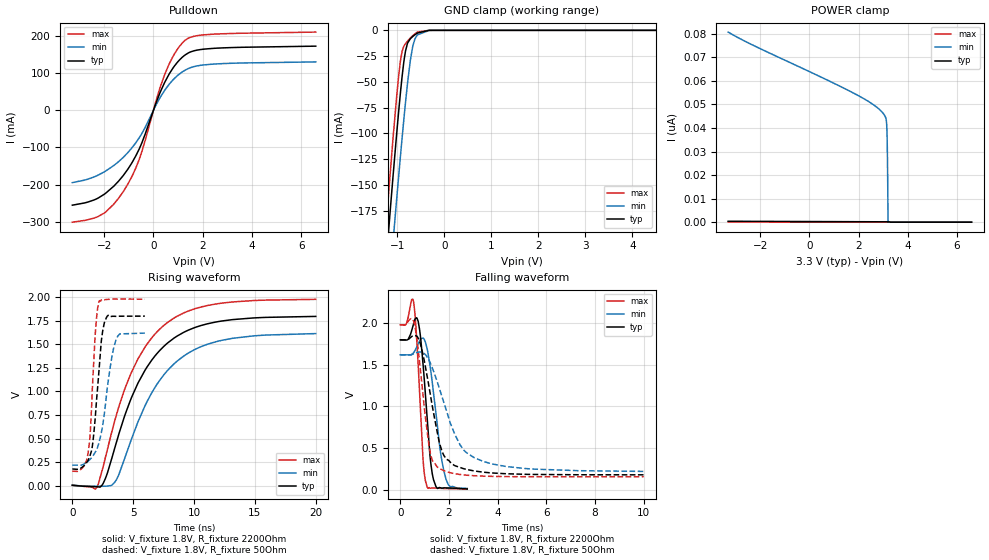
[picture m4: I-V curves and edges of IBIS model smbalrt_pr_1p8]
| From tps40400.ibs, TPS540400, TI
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|   smbalrt_pr_1p8 Model
[Model]   smbalrt_pr_1p8
Model_type   Open_sink
Polarity   Inverting
Vmeas = 1.65
Vref = 3.3
Cref = 2pF
Rref = 2200
|   typ   min   max
|   (nom PVT)   (fast PVT)   (slow PVT)
C_comp   1.150e-12   1.129e-12   1.173e-12
| Where nom  PVT is Nominal Process, 3.3V, 25C
|   Fast PVT is Strong Process,  3.4V, -40C
|   Slow PVT is Weak Process,   3.2V, 125C
[Voltage Range]   3.3   3.2   3.4
|Junction Temperature
[Temperature Range]   25   125   -40
[Pullup Reference]   3.3   3.2   3.4
[Pulldown Reference]   0   0   0
[Power Clamp Reference]   3.3   3.2   3.4
[GND Clamp Reference]   0   0   0
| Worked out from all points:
|   slope of the pulldown table from 0 to 0.495 V, typ, clamps not added: 6.2 ohm
|   GND clamp passes 1 mA (typ) near -0.42 V on its own axis
|   falling waveform, V_fixture 1.8V, R_fixture 2200Ohm: 20-80 % time 282ps typ, 406ps min, 210ps max; typ from 1.8 V to 0.007 V
|   rising waveform, V_fixture 1.8V, R_fixture 2200Ohm: 20-80 % time 3.8ns typ, 3.95ns min, 3.71ns max; typ from 0.004 V to 1.8 V
|   falling waveform, V_fixture 1.8V, R_fixture 50Ohm: 20-80 % time 636ps typ, 1.08ns min, 423ps max; typ from 1.8 V to 0.177 V
|   rising waveform, V_fixture 1.8V, R_fixture 50Ohm: 20-80 % time 619ps typ, 942ps min, 438ps max; typ from 0.177 V to 1.8 V
[Pulldown]
|   Voltage   I(typ)   I(min)   I(max)
-3.3V     -255.3mA   -194.7mA   -301.1mA
-2.41V    -241.1mA   -179.3mA   -289.8mA
-2.001V   -225.9mA   -165.7mA   -276.5mA
-1.221V   -174.9mA   -126.2mA   -218mA
-861.6mV  -139.6mA   -99.81mA   -175.9mA
-576.8mV  -103.8mA   -73.77mA   -131.6mA
148.5mV   27.58mA    19.62mA    35.46mA
460.4mV   75.5mA     53.98mA    96.63mA
858mV     119.4mA    85.93mA    152.1mA
1.293V    149mA      108mA      188.4mA
2.422V    166.3mA    124mA      204.5mA
6.597V    172.3mA    129.9mA    210.1mA
[GND Clamp]
|   Voltage   I(typ)   I(min)   I(max)
-3.3V     -1.486A    -1.512A    -1.478A
-1.277V   -244.6mA   -306.4mA   -209.5mA
-1.127V   -159.8mA   -223.3mA   -123.2mA
-1.092V   -140.4mA   -204mA     -103.6mA
-1.019V   -101.2mA   -164.7mA   -65.03mA
-940.4mV  -62.25mA   -124.1mA   -30.94mA
-903mV    -45.55mA   -105.3mA   -20.73mA
-828.3mV  -20.01mA   -69.82mA   -12.85mA
-724mV    -8.058mA   -28.57mA   -7.408mA
-672.8mV  -5.897mA   -15.15mA   -5.152mA
-570.4mV  -2.564mA   -4.36mA    -1.648mA
6.597V    0A         0A         0A
[POWER Clamp]
|   Voltage   I(typ)   I(min)   I(max)
-3.3V     396.6pA    80.72nA    94.42pA
1.782V    213.1pA    54.91nA    23.02pA
2.504V    185.7pA    50.61nA    12.87pA
2.998V    163.7pA    46.27nA    5.93pA
3.116V    156.8pA    43.98nA    4.264pA
3.148V    154.5pA    40.78nA    3.813pA
3.161V    153.5pA    36.79nA    3.633pA
3.174V    152.5pA    29.42nA    3.452pA
3.186V    151.4pA    17.72nA    3.272pA
3.199V    150.2pA    1.198nA    3.091pA
3.206V    149.5pA    0A         3.001pA
6.597V    0A         0A         0A
[Ramp]
R_load = 2200
|   typ   min   max
dV/dt_r   1.0757/3.80042e-09   0.965617/3.94989e-09   1.18472/3.70414e-09
dV/dt_f   1.07751/2.81407e-10   0.968767/4.0919e-10   1.18587/2.09469e-10
[Falling Waveform]
V_fixture = 1.8V
V_fixture_min = 1.62V
V_fixture_max = 1.98V
R_fixture = 2200Ohm
|   Time   V(typ)   V(min)   V(max)
0s        1.8V       1.62V      1.98V
550ps     1.994V     1.646V     2.251V
638ps     2.062V     1.69V      1.985V
792ps     1.929V     1.785V     1.186V
948ps     1.469V     1.82V      320.5mV
1.11ns    843.9mV    1.686V     27.62mV
1.366ns   119.3mV    1.163V     18.94mV
1.628ns   22.38mV    497.1mV    15.08mV
1.886ns   19.78mV    119.3mV    11.68mV
2.752ns   7.052mV    13.68mV    4.393mV
[Rising Waveform]
V_fixture = 1.8V
V_fixture_min = 1.62V
V_fixture_max = 1.98V
R_fixture = 2200Ohm
|   Time   V(typ)   V(min)   V(max)
0s        4.152mV    5.263mV    3.546mV
2.01ns    -11.76mV   -6.398mV   -19.87mV
2.54ns    25.19mV    -6.273mV   205.2mV
3.44ns    379.2mV    29.28mV    667.3mV
4.366ns   765.3mV    313.6mV    1.046V
5.364ns   1.08V      666.8mV    1.338V
7.78ns    1.509V     1.217V     1.729V
9.542ns   1.652V     1.409V     1.855V
11.79ns   1.737V     1.528V     1.929V
20ns      1.797V     1.615V     1.978V
[Falling Waveform]
V_fixture = 1.8V
V_fixture_min = 1.62V
V_fixture_max = 1.98V
R_fixture = 50Ohm
|   Time   V(typ)   V(min)   V(max)
0s        1.8V       1.62V      1.98V
552ps     1.851V     1.632V     2.022V
826ps     1.754V     1.654V     1.444V
1.192ns   1.22V      1.549V     506.4mV
1.344ns   960.9mV    1.442V     334.5mV
1.606ns   564mV      1.218V     254.3mV
1.906ns   363.6mV    941.4mV    215.2mV
2.458ns   265.5mV    536.9mV    180.6mV
3.414ns   208.7mV    337.9mV    161.2mV
10ns      176.7mV    217.9mV    153.3mV
[Rising Waveform]
V_fixture = 1.8V
V_fixture_min = 1.62V
V_fixture_max = 1.98V
R_fixture = 50Ohm
|   Time   V(typ)   V(min)   V(max)
0s        176.7mV    217.9mV    153.3mV
1.294ns   268.2mV    259.8mV    345.2mV
1.482ns   330.4mV    282.4mV    583.7mV
1.72ns    497.1mV    320mV      1.216V
1.986ns   902.7mV    381.2mV    1.776V
2.208ns   1.25V      465.7mV    1.959V
2.392ns   1.545V     567.2mV    1.971V
2.67ns    1.745V     803.8mV    1.974V
3.576ns   1.798V     1.542V     1.981V
5.958ns   1.8V       1.62V      1.98V
